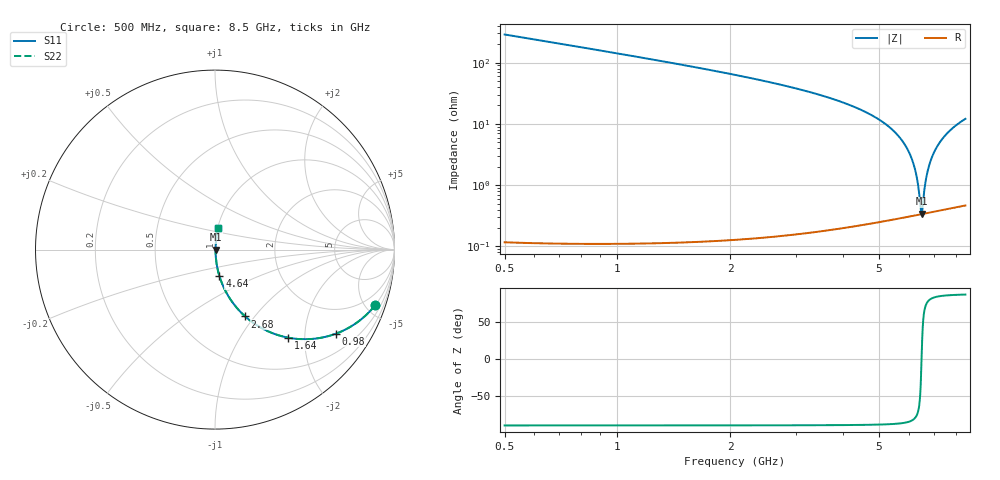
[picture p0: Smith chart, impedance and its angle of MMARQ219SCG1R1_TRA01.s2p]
! MMARQ219SCG1R1_TRA01  S-PARAMETER MODEL  ( General Type )
! Model Generated by TAIYO YUDEN Corporation (http://www.ty-top.com)
! Version 1.0
! TAIYO YUDEN Control No. 180601
! Copyright(c) 2018 TAIYO YUDEN CO.,LTD. All Rights Reserved.
! Product Description (link to TY-COMPAS)
! https://ds.yuden.co.jp/TYCOMPAS/or/detail?pn=MMARQ219SCG1R1BTRA01&u=M
! Products Name : Multilayer Ceramic Capacitors
! Characteristics :
!  Capacitance : 1.1 pF , Rated Voltage : 250V , TCC : CG / C0G
!  Case Size : 2.0 x 1.25 / 0.079 x 0.049 [mm/inch] , Thickness : 0.85 / 0.033 [mm/inch]
!  (Conditions: Temperature = 25 degC , DC Bias Current/Voltage = 0A / 0V)
! External Node Assignments :
!  1  o---| |---o  2
! GND o---------o GND
! Frequency Range : 500MHz  -  8500MHz  [ 401 STEP ]
# MHz S RI R 50
! Freq[MHz].  S11 Real  S11 Imag  S21 Real  S21 Imag  S12 Real  S12 Imag  S22 Real  S22 Imag
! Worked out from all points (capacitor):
!   401 points, 500 MHz to 8.5 GHz, reference 50 ohm
!   read as one part in series: C = 1.1 pF near 540 MHz
!   lowest |Z| = 341 mohm at 6.5 GHz (marker M1)
!   series resonance near 6.492 GHz, so ESL is about 550 pH
!   S11 on the Smith chart (normalised r, x): 500 MHz: 1.00, -5.76; 980 MHz: 1.00, -2.89; 1.64 GHz: 1.00, -1.65; 2.68 GHz: 1.00, -0.90; 4.64 GHz: 1.00, -0.30; 8.5 GHz: 1.01, +0.24
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500  0.8923 -0.3098  0.1077 0.3098  0.1077 0.3098  0.8923 -0.3098
980  0.6758 -0.4677  0.3242 0.4677  0.3242 0.4677  0.6758 -0.4677
1640  0.4061 -0.4904  0.5939 0.4904  0.5939 0.4904  0.4061 -0.4904
1840  0.344 -0.4742  0.656 0.4742  0.656 0.4742  0.344 -0.4742
2680  0.168 -0.3722  0.832 0.3722  0.832 0.3722  0.168 -0.3722
3180  0.108 -0.308  0.892 0.308  0.892 0.308  0.108 -0.308
4500  0.0292 -0.1617  0.9708 0.1617  0.9708 0.1617  0.0292 -0.1617
4640  0.0248 -0.1483  0.9752 0.1483  0.9752 0.1483  0.0248 -0.1483
5340  0.0102 -0.0864  0.9898 0.0864  0.9898 0.0864  0.0102 -0.0864
5840  0.00516 -0.0468  0.9948 0.0468  0.9948 0.0468  0.00516 -0.0468
6060  0.00402 -0.0304  0.996 0.0304  0.996 0.0304  0.00402 -0.0304
6220  0.00355 -0.0189  0.9965 0.0189  0.9965 0.0189  0.00355 -0.0189
6340  0.00337 -0.0105  0.9966 0.0105  0.9966 0.0105  0.00337 -0.0105
6460  0.00334 -0.00218  0.9967 0.00218  0.9967 0.00218  0.00334 -0.00218
6500  0.00336 0.000546  0.9966 -0.000546  0.9966 -0.000546  0.00336 0.000546
6540  0.00339 0.00325  0.9966 -0.00325  0.9966 -0.00325  0.00339 0.00325
6640  0.00354 0.00995  0.9965 -0.00995  0.9965 -0.00995  0.00354 0.00995
6760  0.00384 0.0179  0.9962 -0.0179  0.9962 -0.0179  0.00384 0.0179
6940  0.0045 0.0294  0.9955 -0.0294  0.9955 -0.0294  0.0045 0.0294
7180  0.00577 0.0444  0.9942 -0.0444  0.9942 -0.0444  0.00577 0.0444
7720  0.01 0.0762  0.99 -0.0762  0.99 -0.0762  0.01 0.0762
8500  0.0189 0.1182  0.9811 -0.1182  0.9811 -0.1182  0.0189 0.1182
